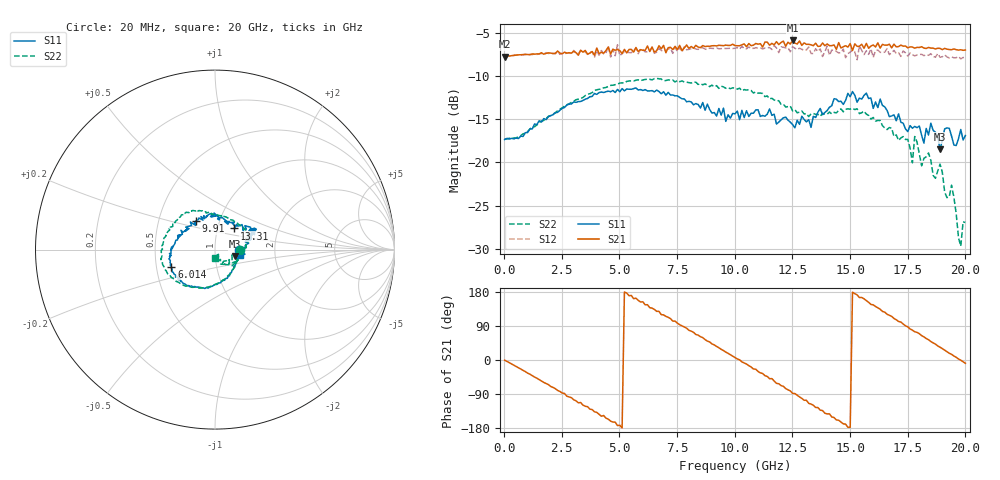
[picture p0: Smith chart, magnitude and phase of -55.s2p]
!Agilent Technologies,N5230A,US43500223,A.07.50.48
!Agilent N5230A: A.07.50.48
!Date: Wednesday, October 07, 2015 13:20:27
!Correction: S11(Full 2 Port(1,2))
!S21(Full 2 Port(1,2))
!S12(Full 2 Port(1,2))
!S22(Full 2 Port(1,2))
!S2P File: Measurements: S11, S21, S12, S22:
# Hz S  RI  R 50
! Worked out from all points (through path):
!   201 points, 20 MHz to 20 GHz, reference 50 ohm
!   highest |S21| = -5.87 dB at 12.51 GHz (marker M1); lowest = -7.7 dB at 20 MHz (marker M2)
!   group delay of S21, straight-line fit = 101 ps
!   lowest |S11| = -18.5 dB at 18.9 GHz (marker M3), VSWR 1.27, Z = 62.6 - j4.61 ohm
!   |S11| at or under -10 dB: start of sweep to end of sweep
!   |S22| runs from -29.7 to -10.3 dB; largest |S21 - S12| = 0.1
!   S11 on the Smith chart (normalised r, x): 20 MHz: 1.31, -0.01; 6.014 GHz: 0.60, -0.12; 9.91 GHz: 0.77, +0.25; 13.31 GHz: 1.20, +0.29; 20 GHz: 1.32, -0.08
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2e7  0.1356 -0.00477  0.4099 -0.00342  0.4093 -0.00487  0.1366 -0.00384
1.8182e9  0.0466 -0.1707  0.2012 -0.3782  0.1945 -0.3865  0.0359 -0.1757
3.4166e9  -0.0927 -0.2088  -0.2102 -0.3817  -0.237 -0.37  -0.1131 -0.2091
4.9151e9  -0.2051 -0.1674  -0.4477 -0.0546  -0.4776 -0.0512  -0.2367 -0.1576
6.014e9  -0.2432 -0.0949  -0.3998 0.1985  -0.3791 0.2473  -0.2849 -0.0945
6.7133e9  -0.2531 -0.0478  -0.2943 0.372  -0.2617 0.3742  -0.301 -0.0504
7.9121e9  -0.2215 0.0365  0.0502 0.4763  0.0906 0.44  -0.2894 0.0359
9.9101e9  -0.1082 0.1587  0.4757 0.0885  0.4549 0.0432  -0.2041 0.1777
1.001e10  -0.0925 0.1673  0.4723 0.052  0.4585 0.0113  -0.2031 0.176
1.14086e10  -0.00906 0.19  0.3611 -0.3424  0.2981 -0.3516  -0.1038 0.2194
1.25075e10  0.0535 0.157  0.0173 -0.5086  -0.015 -0.4684  -0.0201 0.1979
1.33067e10  0.1073 0.1181  -0.2129 -0.4303  -0.2223 -0.3654  0.0459 0.1856
1.34066e10  0.1204 0.1403  -0.2326 -0.4135  -0.235 -0.357  0.0605 0.1821
1.54046e10  0.2093 0.1088  -0.4545 0.1229  -0.4552 0.1277  0.1788 0.0693
1.67033e10  0.1761 0.0537  -0.2272 0.4272  -0.1596 0.3899  0.1588 -0.0109
1.76024e10  0.1631 0.0104  0.0652 0.4626  0.0853 0.422  0.0957 -0.0737
1.85015e10  0.167 -0.025  0.3026 0.3456  0.3171 0.2852  0.06 -0.0834
1.89011e10  0.1132 -0.0363  0.3805 0.2542  0.3657 0.1783  0.0528 -0.0822
1.92008e10  0.1555 -0.0298  0.4205 0.1685  0.3958 0.1024  0.0294 -0.0551
1.94006e10  0.1371 -0.0365  0.4344 0.1161  0.4051 0.0536  0.0301 -0.0673
1.98002e10  0.1551 0.00246  0.4495 -0.00504  0.3939 -0.0568  0.0193 -0.0264
2e10  0.1404 -0.0278  0.4429 -0.0672  0.3909 -0.1173  -0.000735 -0.0448
